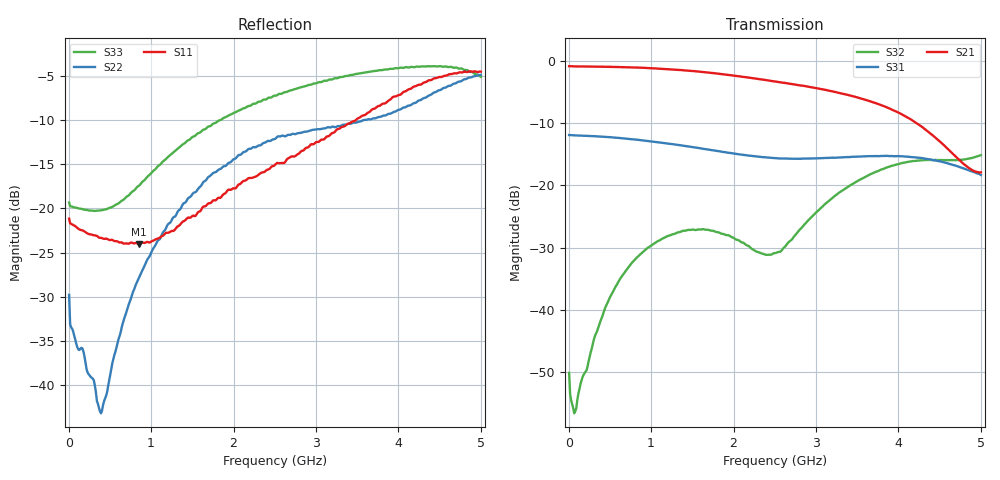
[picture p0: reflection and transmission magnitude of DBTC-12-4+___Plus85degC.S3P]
! Mini-Circuits
! S3P DATA File Format
! Type: Directional Coupler
! Model:DBTC-12-4+
! PINOUT: IN PORT=PORT1 , OUT PORT=PORT2 , COUPLED PORT=PORT3
! TEST CONDITIONS: INPUT POWER = 0 dBm @ Temperature = + 85 deg C
! 401 Frequency points
! All S Parameters are in dB deg format
# MHz S DB R 50
!FREQ	MAG(S11)PHS(S11)MAG(S12)PHS(S12)MAG(S13)PHS(S13)
!	MAG(S21)PHS(S21)MAG(S22)PHS(S22)MAG(S23)PHS(S23)
!	MAG(S31)PHS(S31)MAG(S32)PHS(S32)MAG(S33)PHS(S33)
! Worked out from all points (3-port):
!   401 points, 5 MHz to 5 GHz, reference 50 ohm
!   strongest paths, dB at 5 MHz, 1.254 GHz, 2.502 GHz, 3.751 GHz, 5 GHz:
!     S21: -0.9, -1.4, -3.3, -7.0, -17.9
!     S31: -11.9, -13.4, -15.6, -15.3, -18.3
!     S32: -50.1, -27.9, -30.9, -17.7, -15.2
!   lowest |S11| = -24.1 dB at 854.1 MHz (marker M1), VSWR 1.13, Z = 49.6 + j6.23 ohm
!   |S11| at or under -10 dB: start of sweep to 3.485 GHz
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5  -21.17 165.9  -0.87 0.7  -11.96 -179.9
   -0.88 0.6  -29.79 134.2  -50.30 44.0
   -11.93 -180.0  -50.08 42.3  -19.35 167.1
79.93  -22.02 166.8  -0.90 -7.4  -12.01 -191.2
       -0.92 -7.4  -34.86 153.2  -58.14 -74.0
       -11.99 -191.3  -56.24 -66.1  -19.91 170.3
392.11  -23.34 128.4  -0.95 -36.0  -12.20 -233.6
        -0.97 -36.0  -43.18 35.1  -41.55 -206.2
        -12.18 -233.7  -41.53 -206.8  -20.23 152.4
854.15  -24.08 90.1  -1.11 -78.7  -12.75 -294.5
        -1.12 -78.5  -27.83 -107.0  -31.40 -292.7
        -12.72 -294.4  -31.26 -292.9  -17.43 125.2
1703.3  -19.42 22.8  -1.90 -157.8  -14.31 -395.5
        -1.92 -157.5  -16.40 -213.3  -27.13 -403.1
        -14.28 -395.3  -27.18 -403.3  -10.73 28.0
2502.5  -15.08 -63.3  -3.30 -231.8  -15.65 -475.9
        -3.33 -231.5  -12.16 -302.3  -31.01 -437.1
        -15.63 -475.9  -30.87 -437.9  -7.26 -73.4
2977.03  -12.72 -115.4  -4.34 -275.8  -15.71 -520.9
         -4.34 -275.6  -11.11 -355.3  -24.75 -445.6
         -15.68 -521.1  -24.68 -445.9  -5.89 -129.9
3551.45  -9.59 -176.4  -6.07 -330.8  -15.40 -579.9
         -6.09 -330.9  -10.14 -423.0  -18.94 -499.9
         -15.37 -580.1  -18.96 -499.9  -4.71 -194.5
4288.21  -5.92 -254.2  -10.57 -402.1  -15.63 -671.1
         -10.64 -401.9  -7.64 -514.8  -16.03 -581.1
         -15.64 -671.1  -15.98 -581.5  -3.95 -271.5
5000  -4.55 -328.1  -17.80 -422.8  -18.38 -790.3
      -17.92 -422.2  -4.91 -603.0  -15.24 -645.2
      -18.34 -790.4  -15.16 -645.5  -5.14 -341.2
